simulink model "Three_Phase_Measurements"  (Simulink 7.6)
settings: Solver=ode23tb  StartTime=0.0  StopTime=0.05  RelTol=1e-3
StopFcn:
  | close all
  | load amplitude_phase.mat
  | plotyy(x(1,:),x(2,:), x(1,:),x(3,:))
  | grid
  | title('Amplitude et Phase de la tension sur la phase A')
  | xlabel('temps')
  | 
  | figure
  | load PhA_et_RMS.mat
  | plotyy(y(1,:),y(2,:), y(1,:),y(3,:))
  | grid
  | title('Amplitude et Phase de la tension sur la phase A')
  | xlabel('temps')
libraries: powerlib x10, powerlib_extras x4

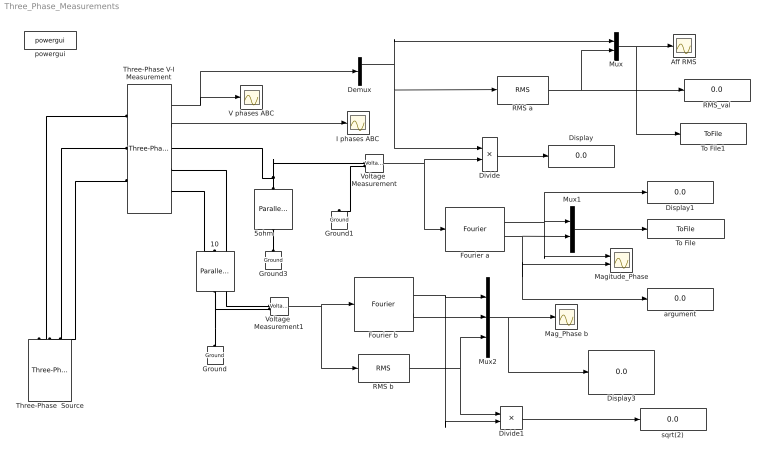
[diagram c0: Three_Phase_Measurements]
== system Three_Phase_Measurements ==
  10 : powerlib/Elements/Parallel RLC Branch  DialogController=POWERSYS.PowerSysDialog  PhysicalDomain=powersysdomain  SubClassName=unknown  LeftPortType=p1  RightPortType=p1  LConnTagsString=a  RConnTagsString=__new0  BranchType=R  Resistance=10  Inductance=1e-3  SetiL0=off  InitialCurrent=0  Capacitance=1e-6  Setx0=off  InitialVoltage=0  Measurements=None
  5ohm : powerlib/Elements/Parallel RLC Branch  DialogController=POWERSYS.PowerSysDialog  PhysicalDomain=powersysdomain  SubClassName=unknown  LeftPortType=p1  RightPortType=p1  LConnTagsString=a  RConnTagsString=__new0  BranchType=R  Resistance=5  Inductance=1e-3  SetiL0=off  InitialCurrent=0  Capacitance=1e-6  Setx0=off  InitialVoltage=0  Measurements=None
  Aff RMS : Scope
  Demux : Demux  Outputs=3
  Display : Display
  Display1 : Display
  Display3 : Display
  Divide : Product  Inputs=*/
  Divide1 : Product  Inputs=/*
  Fourier a : powerlib_extras/Measurements/Fourier  DialogController=POWERSYS.PowerSysDialog  SystemSampleTime=-1  f1=60  n=1
  Fourier b : powerlib_extras/Measurements/Fourier  DialogController=POWERSYS.PowerSysDialog  SystemSampleTime=-1  f1=60  n=1
  Ground : powerlib/Elements/Ground  DialogController=POWERSYS.PowerSysDialog  PhysicalDomain=powersysdomain  SubClassName=unknown  LeftPortType=p1  RightPortType=p1  LConnTagsString=a
  Ground1 : powerlib/Elements/Ground  DialogController=POWERSYS.PowerSysDialog  PhysicalDomain=powersysdomain  SubClassName=unknown  LeftPortType=p1  RightPortType=p1  LConnTagsString=a
  Ground3 : powerlib/Elements/Ground  DialogController=POWERSYS.PowerSysDialog  PhysicalDomain=powersysdomain  SubClassName=unknown  LeftPortType=p1  RightPortType=p1  LConnTagsString=a
  I phases ABC : Scope
  Mag_Phase b : Scope
  Magitude_Phase : Scope  NumInputPorts=2
  Mux : Mux  Inputs=2
  Mux1 : Mux  Inputs=2
  Mux2 : Mux  Inputs=3
  RMS a : powerlib_extras/Measurements/RMS  DialogController=POWERSYS.PowerSysDialog  SystemSampleTime=-1  f1=60
  RMS b : powerlib_extras/Measurements/RMS  DialogController=POWERSYS.PowerSysDialog  SystemSampleTime=-1  f1=60
  RMS_val : Display
  Three-Phase V-I Measurement : powerlib/Measurements/Three-Phase V-I Measurement  DialogController=POWERSYS.PowerSysDialog  SystemSampleTime=-1  VoltageMeasurement=phase-to-ground  SetLabelV=off  LabelV=Vabc  Vpu=off  VpuLL=off  CurrentMeasurement=yes  SetLabelI=off  LabelI=Iabc  Ipu=off  Pbase=100e6  Vbase=500e3  OutputType=Complex  PhasorSimulation=off  PSBequivalent=0
  Three-Phase  Source : powerlib/Electrical Sources/Three-Phase Source  DialogController=POWERSYS.PowerSysDialog  SystemSampleTime=-1  Voltage=25e3  PhaseAngle=0  Frequency=60  InternalConnection=Yg  SpecifyImpedance=off  Resistance=1  Inductance=10e-3  ShortCircuitLevel=100e6  BaseVoltage=25e3  XRratio=7
  To File : ToFile  Filename=amplitude_phase  MatrixName=x
  To File1 : ToFile  Filename=PhA_et_RMS  MatrixName=y
  V phases ABC : Scope
  Voltage  Measurement : powerlib/Measurements/Voltage Measurement  DialogController=POWERSYS.PowerSysDialog  SystemSampleTime=-1  PhasorSimulation=off  OutputType=Complex  PSBequivalent=0
  Voltage  Measurement1 : powerlib/Measurements/Voltage Measurement  DialogController=POWERSYS.PowerSysDialog  SystemSampleTime=-1  PhasorSimulation=off  OutputType=Complex  PSBequivalent=0
  argument : Display
  powergui : powerlib/powergui  SystemSampleTime=-1  SimulationMode=Continuous  SampleTime=0  frequency=60  SPID=off  DisableSnubberDevices=off  DisableRonSwitches=off  DisableVfSwitches=off  SwTol=0  Interpol=off  frequencyindice=60  echomessages=off  HookPort=off  DisplayEquations=off  FunctionMessages=off  EnableUseOfTLC=off  x0status=blocks  RestoreLinks=warning  ResistiveCurrentMeasurement=off  Frange=[0:2:500]  Ylog=off  Xlog=on  ShowGrid=off  save=off  variable=ZData  structure=ScopeData1  ZoomFFT=off  StartTime=0.0  cycles=1  DisplayStyle=1  fundamental=10  FreqAxis=off  MaxFrequency=100  frequencyindicesteady=60  RmsSteady=1  display=off  Ts=0  methode=off
  sqrt(2) : Display
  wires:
  Three-Phase V-I Measurement/1 -> V phases ABC/1, Demux/1
  Three-Phase V-I Measurement/2 -> I phases ABC/1
  Demux/1 -> RMS a/1, Divide/1, Mux/1
  RMS a/1 -> RMS_val/1, Mux/2
  Voltage  Measurement/1 -> Divide/2, Fourier a/1
  Divide/1 -> Display/1
  Mux/1 -> Aff RMS/1, To File1/1
  Fourier a/1 -> Mux1/1, Magitude_Phase/1, Display1/1
  Fourier a/2 -> Mux1/2, Magitude_Phase/2, argument/1
  Mux1/1 -> To File/1
  Voltage  Measurement1/1 -> Fourier b/1, RMS b/1
  RMS b/1 -> Mux2/3, Divide1/1
  Fourier b/2 -> Mux2/2
  Fourier b/1 -> Mux2/1, Divide1/2
  Mux2/1 -> Mag_Phase b/1, Display3/1
  Divide1/1 -> sqrt(2)/1
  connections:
  Three-Phase V-I Measurement/LConn3 -- Three-Phase  Source/RConn3
  Three-Phase V-I Measurement/LConn2 -- Three-Phase  Source/RConn2
  Three-Phase V-I Measurement/RConn3 -- 10/RConn1
  5ohm/LConn1 -- Ground3/LConn1
  Three-Phase V-I Measurement/LConn1 -- Three-Phase  Source/RConn1
  5ohm/RConn1 -- Three-Phase V-I Measurement/RConn1 -- Voltage  Measurement/LConn1
  Voltage  Measurement/LConn2 -- Ground1/LConn1
  Three-Phase V-I Measurement/RConn2 -- Voltage  Measurement1/LConn1
  10/LConn1 -- Ground/LConn1 -- Voltage  Measurement1/LConn2
